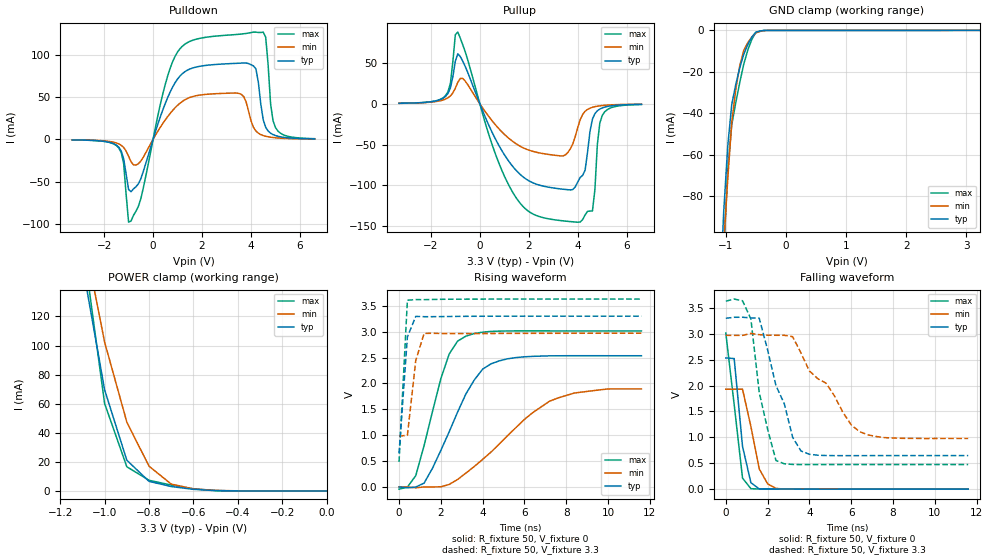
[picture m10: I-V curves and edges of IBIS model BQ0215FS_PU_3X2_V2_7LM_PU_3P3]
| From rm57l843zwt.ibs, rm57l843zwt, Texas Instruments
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|   Model Cell PD_3X2_V2_7LM_PU_3P3
|BQ0215FS_PU_3X2_V2_7LM_PU_3P3
[Model]   BQ0215FS_PU_3X2_V2_7LM_PU_3P3
Model_type   I/O
Polarity   Non-Inverting
Enable   Active-Low
Vinl =  1.25
Vinh =  1.65
Cref =  15.0001pF
Rref =  101.0000M
Vref =  0V
Vmeas =  1.65
C_comp   1.2p   1.2p   1.2p
[Model Spec]
Vinl   1.25   1.12   1.38
Vinh   1.65   1.45   1.75
[Temperature Range]   25   155   -40
[Voltage Range]   3.3   2.97   3.63
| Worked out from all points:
|   slope of the pulldown table from 0 to 0.495 V, typ, clamps not added: 11.8 ohm
|   slope of the pullup table from 0 to 0.495 V, typ, clamps not added: 14.3 ohm
|   GND clamp passes 1 mA (typ) near -0.50 V on its own axis
|   POWER clamp passes 1 mA (typ) near -0.59 V on its own axis
|   rising waveform, R_fixture 50, V_fixture 0: 20-80 % time 1.77ns typ, 3.14ns min, 1.22ns max; typ from 0 V to 2.54 V
|   rising waveform, R_fixture 50, V_fixture 3.3: 20-80 % time 283ps typ, 393ps min, 242ps max; typ from 0.649 V to 3.3 V
|   falling waveform, R_fixture 50, V_fixture 0: 20-80 % time 466ps typ, 593ps min, 516ps max; typ from 2.53 V to 0 V
|   falling waveform, R_fixture 50, V_fixture 3.3: 20-80 % time 1.14ns typ, 2.11ns min, 754ps max; typ from 3.3 V to 0.648 V
[POWER_clamp]
|   voltage   I(typ)   I(min)   I(max)
-3.3V     2.375A     2.63A      3.153A
-1.1V     156mA      180.2mA    173.4mA
-1.067V   127.2mA    154.3mA    135.7mA
-1.033V   98.42mA    128.4mA    97.93mA
-1V       69.62mA    102.5mA    60.21mA
-900mV    21.14mA    47.42mA    16.63mA
-800mV    6.589mA    17.01mA    7.329mA
-700mV    3.011mA    4.694mA    4.008mA
-600mV    1.098mA    1.411mA    1.442mA
-500mV    196.6uA    363.8uA    217.1uA
0V        429.9pA    12.78nA    319.2pA
[Pulldown]
|   voltage   I(typ)   I(min)   I(max)
-3.3V     -560.7uA   -504.5uA   -563.6uA
-1.4V     -9.199mA   -5.273mA   -10.11mA
-1.2V     -22.91mA   -9.491mA   -28.67mA
-1V       -59mA      -19.85mA   -97.49mA
-900mV    -61.64mA   -26.24mA   -96.13mA
1V        71.11mA    40.13mA    102.9mA
3.5V      89.74mA    54.24mA    123.8mA
4.2V      83.16mA    9.923mA    126.4mA
4.6V      14.26mA    3.714mA    120.5mA
4.8V      7.317mA    2.617mA    42.02mA
5V        4.531mA    1.939mA    13.99mA
6.6V      631.1uA    487.2uA    853.6uA
[Pullup]
|   voltage   I(typ)   I(min)   I(max)
-3.3V     614.6uA    591.9uA    551.1uA
-1.4V     9.028mA    5.738mA    10.01mA
-900mV    61.32mA    26.24mA    87.8mA
500mV     -34.85mA   -20.79mA   -49.88mA
1.4V      -78.76mA   -47.33mA   -111.2mA
3.4V      -104.6mA   -63.81mA   -143.4mA
4V        -95.71mA   -29.08mA   -145mA
4.3V      -81.25mA   -9.188mA   -136.1mA
4.6V      -18.8mA    -4.29mA    -131.2mA
4.8V      -8.576mA   -2.945mA   -49.93mA
5V        -5.064mA   -2.148mA   -14.33mA
6.6V      -672.1uA   -541.9uA   -866.9uA
[GND_clamp]
|   voltage   I(typ)   I(min)   I(max)
-3.3V     -1.951A    -1.627A    -3.261A
-1.1V     -130.1mA   -138.8mA   -166.7mA
-1.033V   -87.46mA   -103.2mA   -108mA
-966.7mV  -55.98mA   -71.78mA   -67.59mA
-900mV    -35.71mA   -44.42mA   -45.59mA
-833.3mV  -26.16mA   -28.61mA   -34.93mA
-766.7mV  -18.1mA    -17.01mA   -25.16mA
-700mV    -11.52mA   -9.614mA   -16.29mA
-633.3mV  -6.852mA   -5.986mA   -9.523mA
-500mV    -890.3uA   -1.251mA   -1.035mA
-300mV    -21.3uA    -25.97uA   -33.69uA
3.233V    -1.13uA    6.932uA    -9.303uA
[Ramp]
| variable   typ   min   max
dV/dt_f   1.620167/1.104998n   1.217056/2.126526n   1.924964/0.7613058n
dV/dt_r   1.545231/1.793198n   1.178735/3.282561n   1.835214/1.194523n
R_load = 50
[Rising Waveform]
R_fixture = 50
V_fixture = 0
V_fixture_min = 0
V_fixture_max = 0
|   time   V(typ)   V(min)   V(max)
0s        87.74uV    249.7uV    -43.27mV
800ps     -2.427mV   -16.7mV    218mV
1.2ns     74.48mV    -535.1uV   800.7mV
2ns       705.9mV    2.73mV     2.09V
2.4ns     1.065V     48.34mV    2.568V
2.8ns     1.445V     143.2mV    2.817V
4ns       2.275V     531.6mV    2.99V
4.8ns     2.436V     831.6mV    3.011V
7.2ns     2.533V     1.656V     3.015V
11.6ns    2.535V     1.893V     3.014V
[Rising Waveform]
R_fixture = 50
V_fixture = 3.3
V_fixture_min = 2.97
V_fixture_max = 3.63
|   time   V(typ)   V(min)   V(max)
0s        648.6mV    982.5mV    484.6mV
400ps     2.898V     997.8mV    3.607V
800ps     3.295V     2.442V     3.62V
1.2ns     3.289V     2.966V     3.619V
11.6ns    3.3V       2.97V      3.63V
[Falling Waveform]
R_fixture = 50
V_fixture = 0
V_fixture_min = 0
V_fixture_max = 0
|   time   V(typ)   V(min)   V(max)
0s        2.534V     1.93V      3.014V
400ps     2.522V     1.93V      1.634V
800ps     826.4mV    1.93V      213.8mV
1.2ns     125.6mV    1.211V     9.514mV
1.6ns     4.561mV    392mV      2.718mV
2ns       7.025mV    103.9mV    3.356mV
2.4ns     2.85mV     14.62mV    1.553mV
2.8ns     4.046mV    1.692mV    540uV
11.6ns    167.4uV    173uV      184.9uV
[Falling Waveform]
R_fixture = 50
V_fixture = 3.3
V_fixture_min = 2.97
V_fixture_max = 3.63
|   time   V(typ)   V(min)   V(max)
0s        3.3V       2.97V      3.63V
800ps     3.32V      2.97V      3.638V
1.2ns     3.307V     3.007V     3.286V
1.6ns     3.301V     2.983V     1.866V
2.4ns     2V         2.972V     554.1mV
3.2ns     999.7mV    2.944V     477.3mV
4ns       673.7mV    2.283V     475.1mV
4.8ns     649.7mV    2.046V     475.7mV
6.4ns     647.6mV    1.111V     475.9mV
11.6ns    648.5mV    979.1mV    475.9mV
